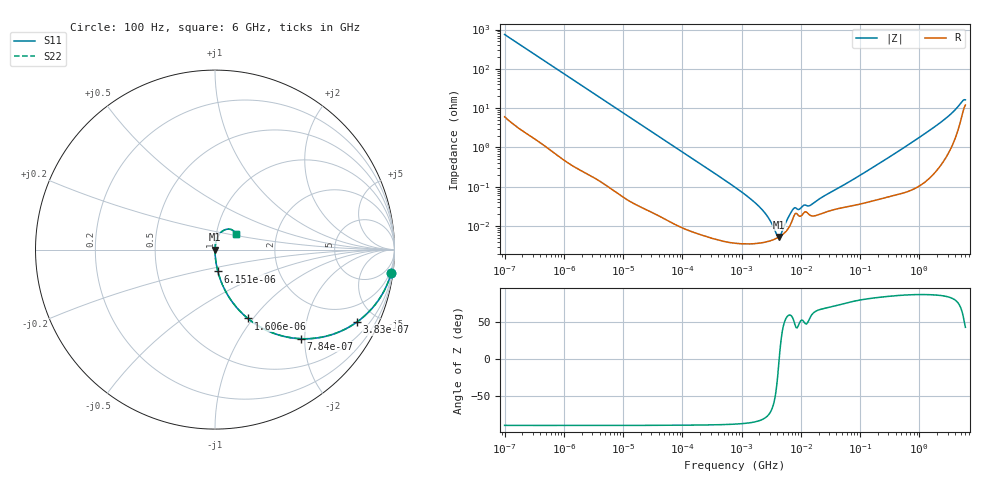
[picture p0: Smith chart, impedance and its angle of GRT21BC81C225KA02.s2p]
!Murata Part Number: GRT21BC81C225KA02
!These Parameters are Measured in Series Mode Connection
!Data Generated on Jun 19, 2026
!  o--ll--o
!Port1  Port2
!  o------o
!Operation Temp=25[degC], DC Bias Voltage=0[V]
!Freq. Start=100[Hz] Stop=6[GHz] 401[Steps]
# Hz S RI R 50
!Freq.(Hz) S11(Real) S11(Imag) S21(Real) S21(Imag) S12(Real) S12(Imag) S22(Real) S22(Imag)
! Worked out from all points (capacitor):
!   401 points, 100 Hz to 6 GHz, reference 50 ohm
!   read as one part in series: C = 2.13 uF near 109 Hz
!   lowest |Z| = 5.27 mohm at 4.246 MHz (marker M1)
!   series resonance near 4.316 MHz, so ESL is about 640 pH
!   S11 on the Smith chart (normalised r, x): 100 Hz: 1, -15; 383 Hz: 1.03, -3.92; 784 Hz: 1.01, -1.92; 1.606 kHz: 1.01, -0.94; 6.151 kHz: 1.00, -0.25; 6 GHz: 1.24, +0.22
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100  0.9814 -0.1311  0.0186 0.1311  0.0186 0.1311  0.9814 -0.1311
205  0.929 -0.2533  0.071 0.2533  0.071 0.2533  0.929 -0.2533
383  0.792 -0.4024  0.208 0.4024  0.208 0.4024  0.792 -0.4024
784  0.4803 -0.4964  0.5197 0.4964  0.5197 0.4964  0.4803 -0.4964
1606  0.1829 -0.3834  0.8171 0.3834  0.8171 0.3834  0.1829 -0.3834
2008  0.1258 -0.3283  0.8742 0.3283  0.8742 0.3283  0.1258 -0.3283
6151  0.0159 -0.1215  0.9841 0.1215  0.9841 0.1215  0.0159 -0.1215
40335  0.000542 -0.019  0.9995 0.019  0.9995 0.019  0.000542 -0.019
774597  3.75e-05 -0.000973  1 0.000973  1 0.000973  3.75e-05 -0.000973
1983483  3.68e-05 -0.000311  1 0.000311  1 0.000311  3.68e-05 -0.000311
2594782  3.95e-05 -0.000193  1 0.000193  1 0.000193  3.95e-05 -0.000193
3394479  4.46e-05 -8.89e-05  1 8.89e-05  1 8.89e-05  4.46e-05 -8.89e-05
4246196  5.24e-05 -6e-06  0.9999 6e-06  0.9999 6e-06  5.24e-05 -6e-06
5311619  6.71e-05 7.98e-05  0.9999 -7.98e-05  0.9999 -7.98e-05  6.71e-05 7.98e-05
7599586  0.000176 0.000221  0.9998 -0.000221  0.9998 -0.000221  0.000176 0.000221
9506416  0.000178 0.000202  0.9998 -0.000202  0.9998 -0.000202  0.000178 0.000202
1.555665e7  0.000181 0.000315  0.9998 -0.000315  0.9998 -0.000315  0.000181 0.000315
3.124326e8  0.000592 0.00567  0.9994 -0.00567  0.9994 -0.00567  0.000592 0.00567
1.431855e9  0.00224 0.0259  0.9978 -0.0259  0.9978 -0.0259  0.00224 0.0259
3.205649e9  0.0119 0.0635  0.9881 -0.0635  0.9881 -0.0635  0.0119 0.0635
5.245841e9  0.0739 0.1144  0.9261 -0.1144  0.9261 -0.1144  0.0739 0.1144
6e9  0.1156 0.087  0.8844 -0.087  0.8844 -0.087  0.1156 0.087
